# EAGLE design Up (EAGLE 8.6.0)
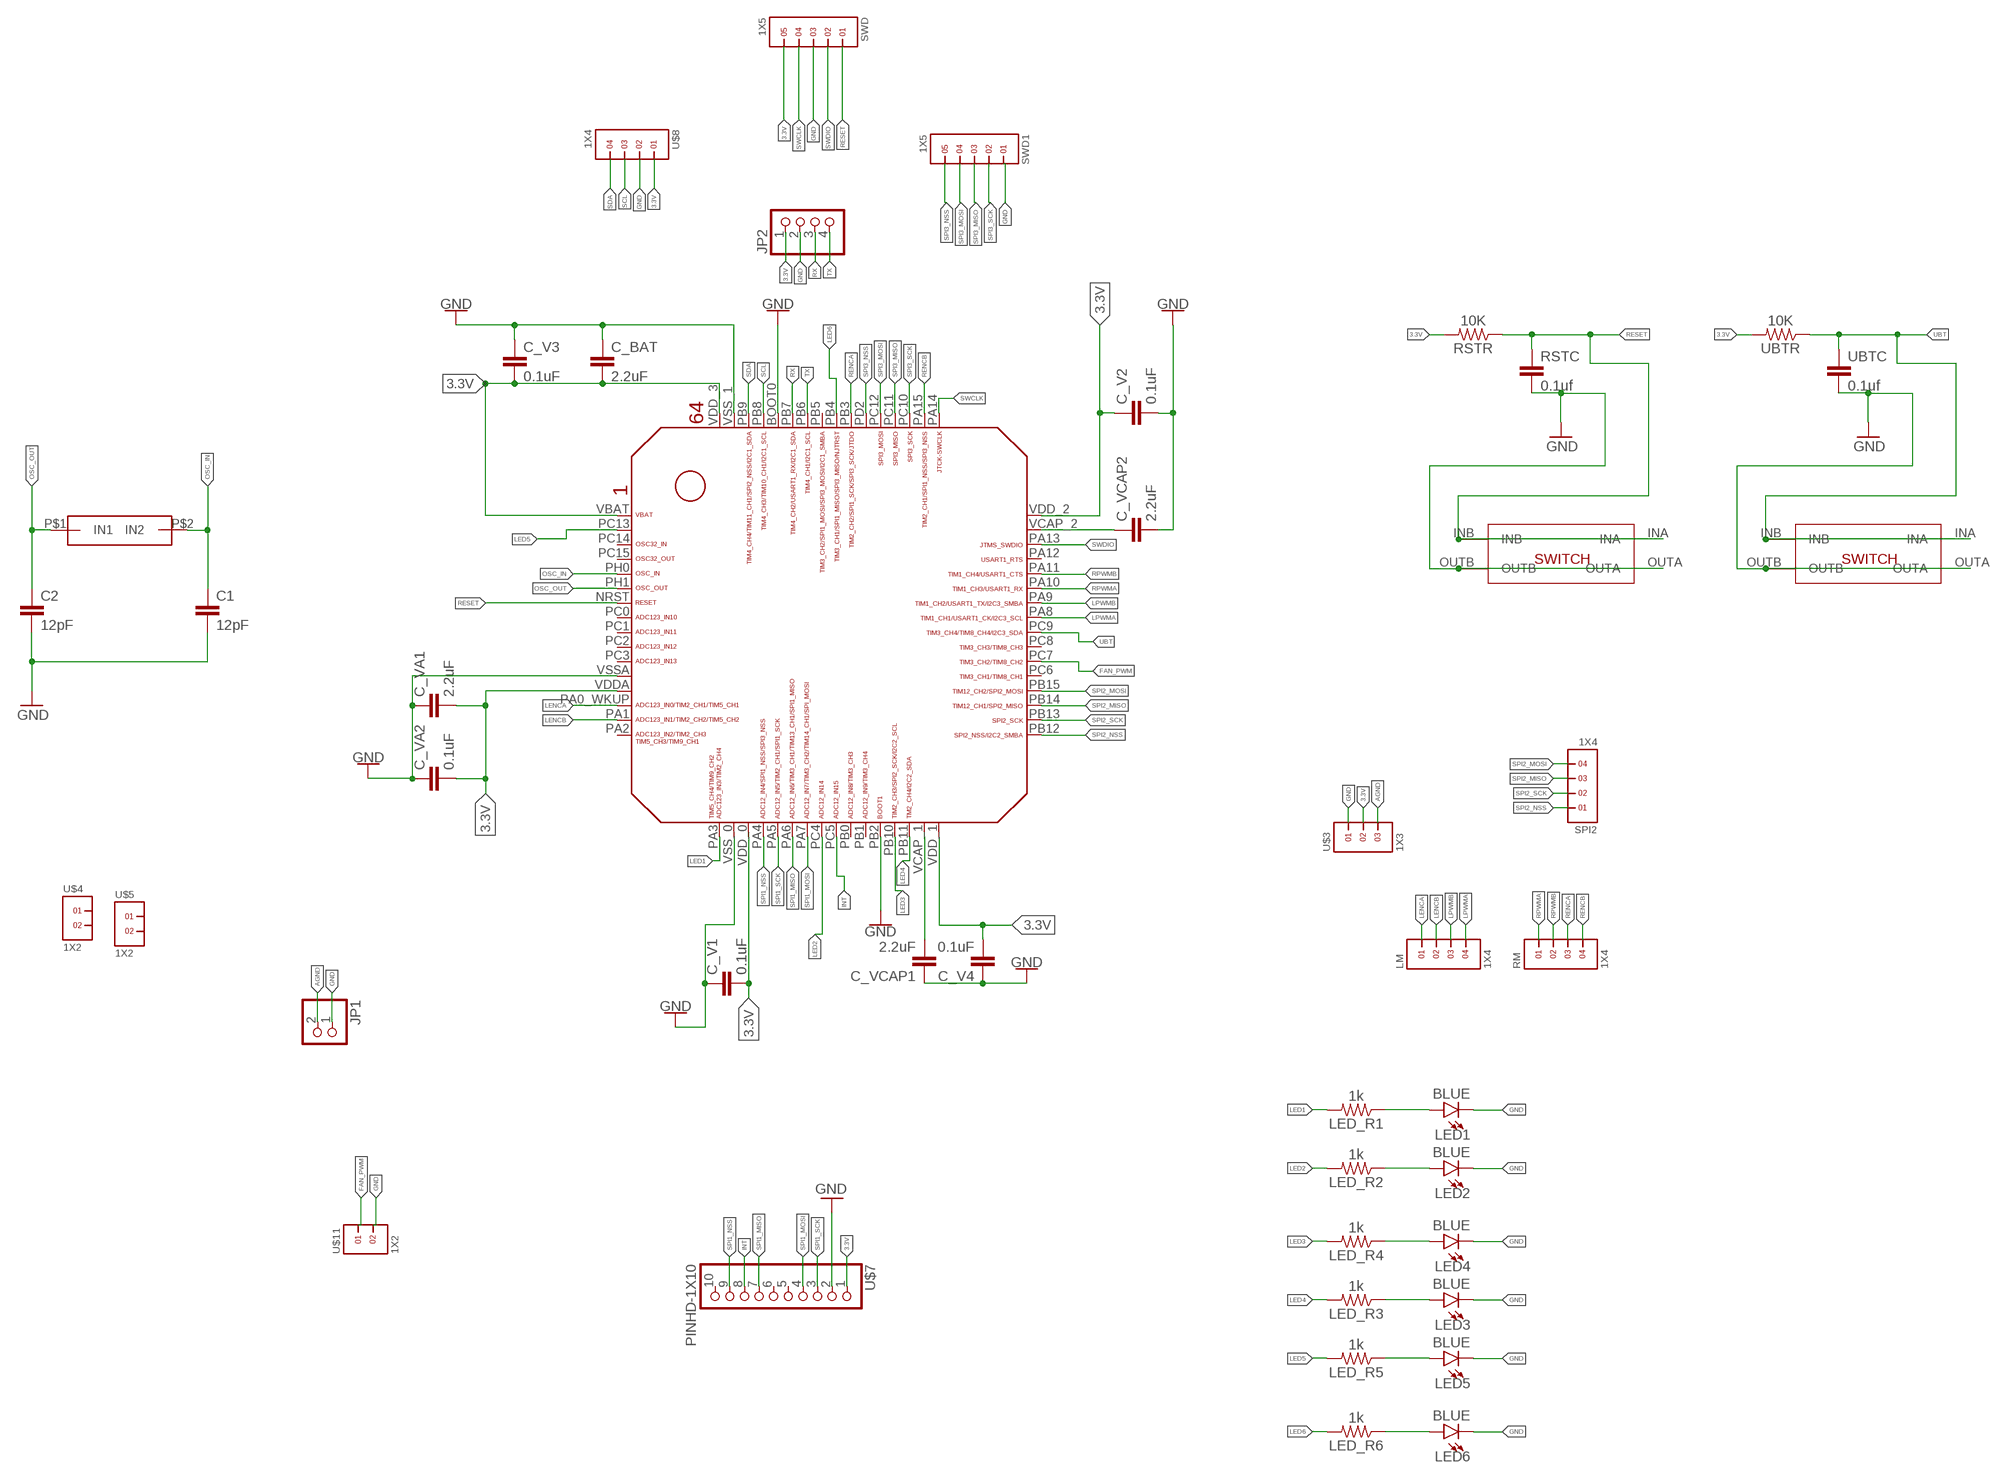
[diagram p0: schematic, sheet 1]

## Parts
C1  12pF  22PF-0603-50V-5%  [0603]
C2  12pF  22PF-0603-50V-5%  [0603]
C_BAT  2.2uF  22UF-0805-6.3V-20%  [0805]
C_V1  0.1uF  22UF-0805-6.3V-20%  [0805]
C_V2  0.1uF  22UF-0805-6.3V-20%  [0805]
C_V3  0.1uF  22UF-0805-6.3V-20%  [0805]
C_V4  0.1uF  22UF-0805-6.3V-20%  [0805]
C_VA1  2.2uF  22UF-0805-6.3V-20%  [0805]
C_VA2  0.1uF  22UF-0805-6.3V-20%  [0805]
C_VCAP1  2.2uF  22UF-0805-6.3V-20%  [0805]
C_VCAP2  2.2uF  22UF-0805-6.3V-20%  [0805]
CX5032GA  OSC  [OSC]
JP1  PINHD-1X2  [1X02]
JP2  PINHD-1X4  [1X04]
LED1  BLUE  LED-BLUE1206  [LED-1206]
LED2  BLUE  LED-BLUE1206  [LED-1206]
LED3  BLUE  LED-BLUE1206  [LED-1206]
LED4  BLUE  LED-BLUE1206  [LED-1206]
LED5  BLUE  LED-BLUE1206  [LED-1206]
LED6  BLUE  LED-BLUE1206  [LED-1206]
LED_R1  1k  0.75OHM-0805-1/4W-1%  [0805]
LED_R2  1k  0.75OHM-0805-1/4W-1%  [0805]
LED_R3  1k  0.75OHM-0805-1/4W-1%  [0805]
LED_R4  1k  0.75OHM-0805-1/4W-1%  [0805]
LED_R5  1k  0.75OHM-0805-1/4W-1%  [0805]
LED_R6  1k  0.75OHM-0805-1/4W-1%  [0805]
LM  1X4  [1X4]
RM  1X4  [1X4]
RSTC  0.1uf  22UF-0805-6.3V-20%  [0805]
RSTR  10K  0.75OHM-0805-1/4W-1%  [0805]
SPI2  1X4  [1X4]
SWD  1X5  [1X5]
SWD1  1X5  [1X5]
U$1  STM32F405/415_LQFP64  [STM32F405/415_LQFP64]
U$3  1X3  [1X3]
U$4  1X2  [1X2]
U$5  1X2  [1X2]
U$7  PINHD-1X10  [1X10-BIG]
U$8  1X4  [1X4]
U$9  4X4X1.5_SMD_SWITCH  [4X4X1.5_SMD_SWITCH]
U$10  4X4X1.5_SMD_SWITCH  [4X4X1.5_SMD_SWITCH]
U$11  1X2  [1X2]
UBTC  0.1uf  22UF-0805-6.3V-20%  [0805]
UBTR  10K  0.75OHM-0805-1/4W-1%  [0805]

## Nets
3.3V: C_BAT.2 C_V1.2 C_V2.1 C_V3.2 C_V4.2 C_VA1.2 C_VA2.2 JP2.1 RSTR.2 SWD.5 U$1.VBAT U$1.VDD_0 U$1.VDD_1 U$1.VDD_2 U$1.VDD_3 U$1.VDDA U$3.2 U$7.1 U$8.1 UBTR.2
AGND: JP1.2 U$3.3
FAN_PWM: U$1.PC7 U$11.1
GND: C1.2 C2.2 C_BAT.1 C_V1.1 C_V2.2 C_V3.1 C_V4.1 C_VA1.1 C_VA2.1 C_VCAP1.1 C_VCAP2.2 JP1.1 JP2.2 LED1.C LED2.C LED3.C LED4.C LED5.C LED6.C RSTC.2 SWD1.1 SWD.3 U$1.BOOT0 U$1.PB2 U$1.VSS_0 U$1.VSS_1 U$1.VSSA U$3.1 U$7.2 U$8.2 U$9.OUTA U$9.OUTB U$10.OUTA U$10.OUTB U$11.2 UBTC.2
INT: U$1.PC5 U$7.8
LED1: LED_R1.2 U$1.PA3
LED2: LED_R2.2 U$1.PC4
LED3: LED_R4.2 U$1.PB10
LED4: LED_R3.2 U$1.PB11
LED5: LED_R5.2 U$1.PC13
LED6: LED_R6.2 U$1.PB4
LENCA: LM.1 U$1.PA0_WKUP(PA0_AKUP)
LENCB: LM.2 U$1.PA1
LPWMA: LM.4 U$1.PA8
LPWMB: LM.3 U$1.PA9
N$1: LED3.A LED_R3.1
N$2: LED4.A LED_R4.1
N$3: LED5.A LED_R5.1
N$4: LED6.A LED_R6.1
N$5: LED2.A LED_R2.1
N$8: LED1.A LED_R1.1
OSC_IN: C1.1 CX5032GA.P$2(IN2) U$1.PH0
OSC_OUT: C2.1 CX5032GA.P$1(IN1) U$1.PH1
RENCA: RM.3 U$1.PB3
RENCB: RM.4 U$1.PA15
RESET: RSTC.1 RSTR.1 SWD.1 U$1.NRST U$9.INA U$9.INB
RPWMA: RM.1 U$1.PA10
RPWMB: RM.2 U$1.PA11
RX: JP2.3 U$1.PB7
SCL: U$1.PB8 U$8.3
SDA: U$1.PB9 U$8.4
SPI1_MISO: U$1.PA6 U$7.7
SPI1_MOSI: U$1.PA7 U$7.4
SPI1_NSS: U$1.PA4 U$7.9
SPI1_SCK: U$1.PA5 U$7.3
SPI2_MISO: SPI2.3 U$1.PB14
SPI2_MOSI: SPI2.4 U$1.PB15
SPI2_NSS: SPI2.1 U$1.PB12
SPI2_SCK: SPI2.2 U$1.PB13
SPI3_MISO: SWD1.3 U$1.PC11
SPI3_MOSI: SWD1.4 U$1.PC12
SPI3_NSS: SWD1.5 U$1.PD2
SPI3_SCK: SWD1.2 U$1.PC10
SWCLK: SWD.4 U$1.PA14
SWDIO: SWD.2 U$1.PA13
TX: JP2.4 U$1.PB6
UBT: U$1.PC9 U$10.INA U$10.INB UBTC.1 UBTR.1
VCAP_1: C_VCAP1.2 U$1.VCAP_1
VCAP_2: C_VCAP2.1 U$1.VCAP_2
Unconnected: U$1.PA2 U$1.PA12 U$1.PB0 U$1.PB1 U$1.PB5 U$1.PC0 U$1.PC1 U$1.PC2 U$1.PC3 U$1.PC6 U$1.PC8 U$1.PC14 U$1.PC15 U$4.1 U$4.2 U$5.1 U$5.2 U$7.5 U$7.6 U$7.10

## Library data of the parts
C1 C2 = SparkFun-Capacitors:22PF: 22pF ceramic capacitors; PROD_ID: CAP-07876; VALUE: 22pF
C_BAT C_V1-C_V4 C_VA1 C_VA2 C_VCAP1 C_VCAP2 RSTC UBTC = SparkFun-Capacitors:22UF: 22µF ceramic capacitors; PROD_ID: CAP-08402; VALUE: 22uF
CX5032GA = Cristal Oscillator:OSC
JP1 = pinhead:PINHD-1X2: PIN HEADER
JP2 = pinhead:PINHD-1X4: PIN HEADER
LED1-LED6 = SparkFun-LED:LED-BLUE: Blue SMD LED; PROD_ID: DIO-09911
LED_R1-LED_R6 RSTR UBTR = SparkFun-Resistors:0.75OHM: 0.75Ω resistor; PROD_ID: RES-08474; VALUE: 0.75
LM RM SPI2 U$8 = headers(2mm):1X4
SWD SWD1 = headers(2mm):1X5
U$1 = STM32F405RG:STM32F405/415_LQFP64
U$3 = headers(2mm):1X3
U$4 U$5 U$11 = headers(2mm):1X2
U$7 = adafruit:PINHD-1X10: Pin header 1x10 0.1" spacing With round pins
U$9 U$10 = 4X4X1.5_SMD_SWITCH:4X4X1.5_SMD_SWITCH

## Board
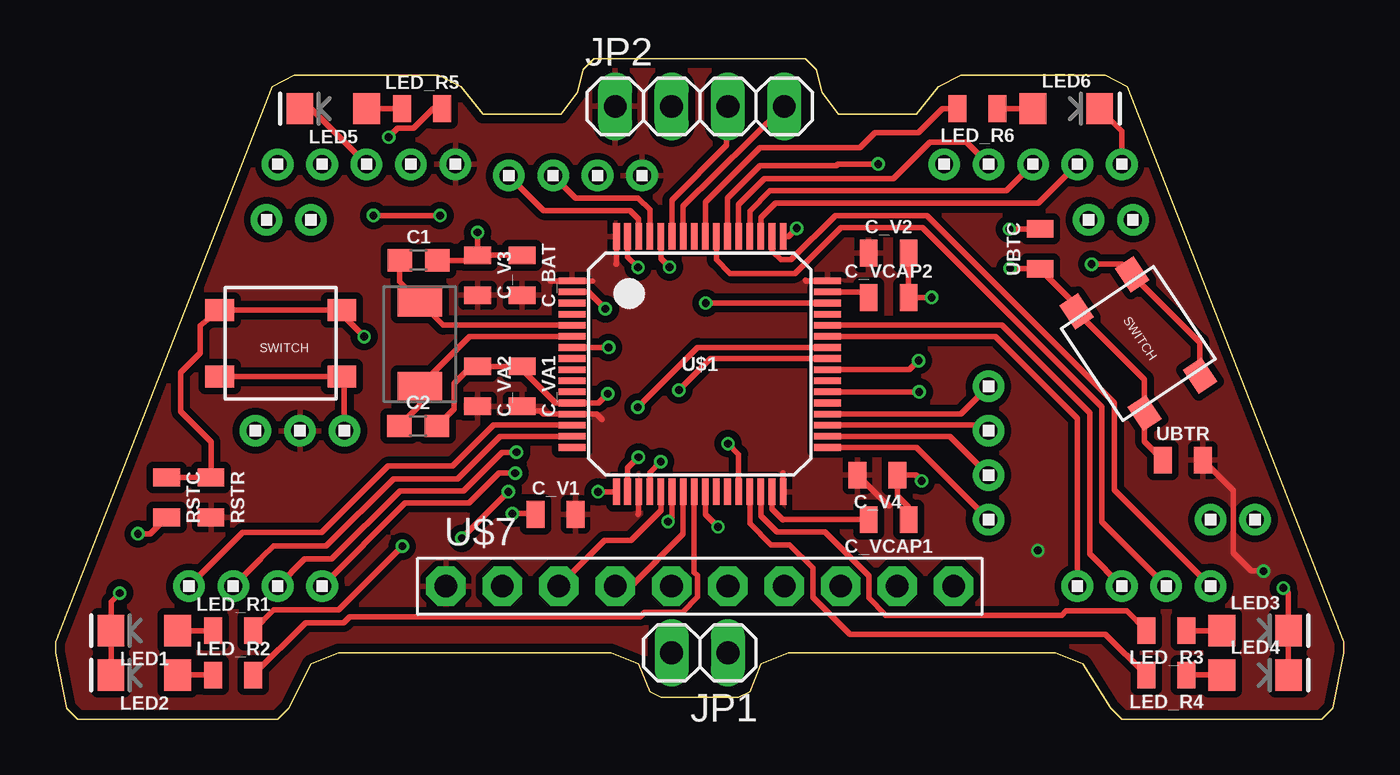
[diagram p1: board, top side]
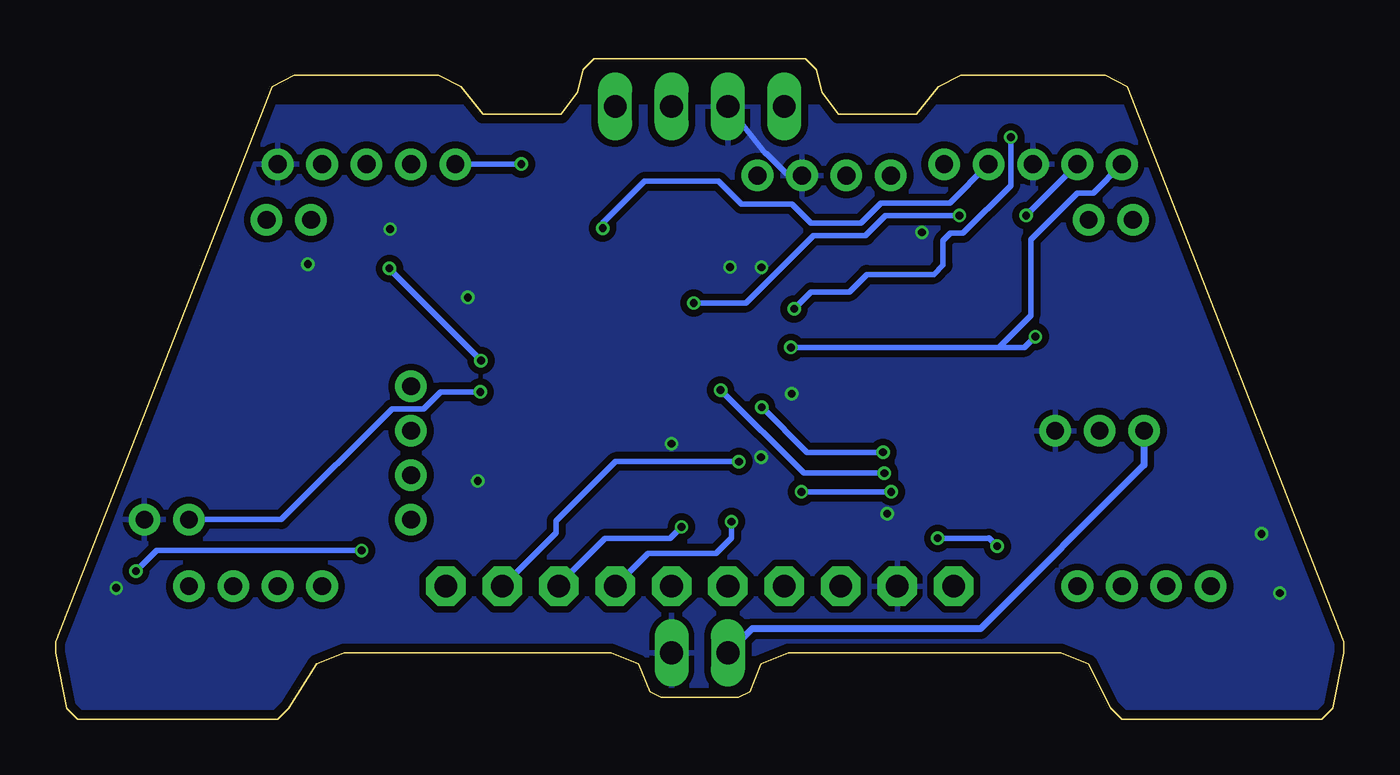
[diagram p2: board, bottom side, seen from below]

Size 58 x 29.75 mm. Coordinates in mm from the lower left corner, seen from the top.
Outline: 47.25,29 40.75,29 39.75,28.5 38.75,27.25 35.25,27.25 34.5,28.25 34.25,29.25 33.75,29.75 24.25,29.75 23.75,29.25 23.5,28.25 22.75,27.25 19.25,27.25 18.25,28.5 17.25,29 10.75,29 9.75,28.5 0,3.5 0,3 0.5,0.5 1,0 10,0 10.5,0.5 11.5,2.5 12.75,3 25,3 26.25,2.5 26.75,1.25 27.25,1 30.75,1 31.25,1.25 31.75,2.5 33,3 45,3 46.25,2.5 47.5,0.5 48,0 57,0 57.5,0.5 58,3 58,3.5 48.25,28.5 47.25,29
Copper layers (1*16): Top 0.035559375mm / dielectric 1.6mm / Bottom 0.035559375mm
Design rules "oshpark-2layer *": minimum track width 6mil, minimum drill 10mil, track to track 6mil, track to pad 6mil, pad to pad 6mil, via to via 6mil, smd to smd 6mil, copper to edge 15mil, drill to drill 6mil, minimum pad ring 5mil, minimum via ring 5mil, stop-mask expansion 2.5mil, vias tented up to drill 12mil, thermal gap 10mil

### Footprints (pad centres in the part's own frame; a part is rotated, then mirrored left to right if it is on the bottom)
0603 = smd 1.1 x 1: 1 -0.85,0; 2 0.85,0
0805 = smd 0.8 x 1.2: 1 -0.9,0; 2 0.9,0
OSC = smd 1.3 x 2: P$1 0,0.1; P$2 3.8,0.1
1X02 = drill 1.016 long: 1 -1.27,0; 2 1.27,0
1X04 = drill 1.016 long: 1 -3.81,0; 2 -1.27,0; 3 1.27,0; 4 3.81,0
LED-1206 = smd 1.2 x 1.4: A -1.5,0; C 1.5,0
1X4 = drill 0.8 pad 1.422: 1 -3,0; 2 -1,0; 3 1,0; 4 3,0
1X5 = drill 0.8 pad 1.422: 1 -4,0; 2 -2,0; 3 0,0; 4 2,0; 5 4,0
STM32F405/415_LQFP64 = smd 0.3 x 1.2: BOOT0 -1.75,5.75; PA3 -3.75,-5.75; PA4 -2.25,-5.75; PA5 -1.75,-5.75; PA6 -1.25,-5.75; PA7 -0.75,-5.75; PA14 3.75,5.75; PA15 3.25,5.75; PB0 0.75,-5.75; PB1 1.25,-5.75; PB2 1.75,-5.75; PB3 0.75,5.75; PB4 0.25,5.75; PB5 -0.25,5.75; PB6 -0.75,5.75; PB7 -1.25,5.75; PB8 -2.25,5.75; PB9 -2.75,5.75; PB10 2.25,-5.75; PB11 2.75,-5.75; PC4 -0.25,-5.75; PC5 0.25,-5.75; PC10 2.75,5.75; PC11 2.25,5.75; PC12 1.75,5.75; PD2 1.25,5.75; VCAP_1 3.25,-5.75; VDD_0 -2.75,-5.75; VDD_1 3.75,-5.75; VDD_3 -3.75,5.75; VSS_0 -3.25,-5.75; VSS_1 -3.25,5.75 | smd 1.2 x 0.3: NRST -5.75,0.75; PA0_WKUP -5.75,-2.75; PA1 -5.75,-3.25; PA2 -5.75,-3.75; PA8 5.75,0.25; PA9 5.75,0.75; PA10 5.75,1.25; PA11 5.75,1.75; PA12 5.75,2.25; PA13 5.75,2.75; PB12 5.75,-3.75; PB13 5.75,-3.25; PB14 5.75,-2.75; PB15 5.75,-2.25; PC0 -5.75,0.25; PC1 -5.75,-0.25; PC2 -5.75,-0.75; PC3 -5.75,-1.25; PC6 5.75,-1.75; PC7 5.75,-1.25; PC8 5.75,-0.75; PC9 5.75,-0.25; PC13 -5.75,3.25; PC14 -5.75,2.75; PC15 -5.75,2.25; PH0 -5.75,1.75; PH1 -5.75,1.25; VBAT -5.75,3.75; VCAP_2 5.75,3.25; VDD_2 5.75,3.75; VDDA -5.75,-2.25; VSSA -5.75,-1.75
1X3 = drill 0.8 pad 1.422: 1 -2,0; 2 0,0; 3 2,0
1X2 = drill 0.8 pad 1.422: 1 -1,0; 2 1,0
1X10-BIG = drill 1.016 pad 1.778 octagon: 1 -11.43,0; 2 -8.89,0; 3 -6.35,0; 4 -3.81,0; 5 -1.27,0; 6 1.27,0; 7 3.81,0; 8 6.35,0; 9 8.89,0; 10 11.43,0
4X4X1.5_SMD_SWITCH = smd 1.3 x 1: INA -2.75,-1.5; INB 2.75,-1.5; OUTA -2.75,1.5; OUTB 2.75,1.5

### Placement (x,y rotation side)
C1  16.34,20.67 0 top
C2  16.32,13.21 0 top
C_BAT  21,20 270 top
C_V1  22.51,9.23 0 top
C_V2  37.5,21 0 top
C_V3  19,20 270 top
C_V4  37,11 180 top
C_VA1  21,15 270 top
C_VA2  19,15 270 top
C_VCAP1  37.5,9 180 top
C_VCAP2  37.5,19 0 top
CX5032GA  16.5,15 90 top
JP1  29,3 180 top
JP2  29,27.61 0 top
LED1  4,4 180 top
LED2  4,2 180 top
LED3  54,4 0 top
LED4  54,2 0 top
LED5  12.5,27.5 180 top
LED6  45.5,27.5 0 top
LED_R1  8,4 0 top
LED_R2  8,2 0 top
LED_R3  50,4 180 top
LED_R4  50,2 180 top
LED_R5  16.5,27.5 0 top
LED_R6  41.5,27.5 180 top
LM  9,6 0 top
RM  49,6 0 top
RSTC  5,10 270 top
RSTR  7,10 270 top
SPI2  42,12 90 top
SWD  14,25 0 top
SWD1  44,25 180 top
U$1  29,16 0 top
U$3  11,13 180 top
U$4  10.5,22.5 0 top
U$5  47.5,22.5 0 top
U$7  29,6 0 top
U$8  23.4,24.49 180 top
U$9  10.14,16.94 180 top
U$10  48.74,16.92 303.8 top
U$11  53,9 0 top
UBTC  44.32,21.19 90 top
UBTR  50.75,11.68 0 top

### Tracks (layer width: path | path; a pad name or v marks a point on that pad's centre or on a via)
3.3V  (via drill 0.35)
  Top 0.254: C_VA1.2 21.21,13.89 21.84,13.89 21.98,13.75 U$1.VDDA 24.36,13.75 24.6,13.51 | 26.22,9.24 26.25,9.27 U$1.VDD_0 | U$1.VDD_1 32.75,11.09 32.74,11.1 | U$1.VDD_2 33.79,19.75 33.76,19.78 | 24.17,19.74 24.16,19.75 U$1.VBAT 22.28,19.75 22.27,19.76 | U$1.VDD_3 25.25,20.51 25.24,20.5 | C_V4.2 37.4,9.7 37.42,9.7 37.51,9.61 37.54,9.61 | UBTR.2 53.01,10.32 53.01,8.59 53.01,7.5 53.83,6.68 v54.38,6.68
  Bottom 0.254: v54.38,6.68 53.45,7.61 v44.22,7.61
  pour Top (isolate 0.305): -4.12,-4.71 62.31,-4.71 62.31,31.86 -4.13,31.86
AGND
  Bottom 0.305: U$3.3 9,11.45 16.36,4.09 26.64,4.09 JP1.2
FAN_PWM  (via drill 0.35)
  Top 0.254: U$1.PC7 v38.88,14.75
  Bottom 0.254: v38.88,14.75 40.66,14.75 41.42,13.99 41.59,13.99 42.85,13.99 47.84,9 U$11.1
GND  (via drill 0.35)
  Top 0.254: C_V2.2 C_VCAP2.2 v39.44,19 | C_VCAP1.1 38.4,9.57 37.9,10.07 C_V4.1 38.73,11 v38.99,10.74 | C2.2 17.93,13.97 17.93,15.13 18.7,15.9 C_VA2.1 C_VA1.1 21,15.75 22.5,14.25 U$1.VSSA 24.44,14.25 v24.86,14.67 | C1.2 18.77,20.67 C_V3.1 | C_V3.1 C_BAT.1 | U$1.VSS_1 25.75,20.83 v26.22,20.36 | U$1.BOOT0 27.25,20.76 v27.64,20.37 | U$1.VSS_0 25.75,11.32 v26.24,11.81 | C_V1.1 21.57,9.27 v20.56,9.27 | U$1.PB2 30.75,11.94 v30.27,12.42 | C_V3.1 v19,21.93 | UBTC.2 v42.95,22.09 v42.94,22.08 | v46.64,20.5 48,20.5 U$10.OUTA 51.52,16.98 U$10.OUTB | U$9.OUTB U$9.OUTA 13,15.16 U$3.1 | RSTC.2 4.26,8.36 v3.71,8.36 | LED2.C LED1.C 2.5,5.3 v2.89,5.69 | LED4.C LED3.C 55.5,5.69 v55.27,5.92 | SWD.3 11.5,27.5 LED5.C | SWD1.1 48,26.5 LED6.C
  Bottom 0.254: JP2.2 26.04,25.48 25.99,25.48 25,24.49 U$8.2
  pour Bottom (isolate 0.305): -0.43,2.98 -0.43,27.57 57.55,27.57 58.44,27.57 58.44,2.81 58.44,-0.99 -0.21,-0.99 -0.44,-0.99 -0.44,2.99
INT  (via drill 0.35)
  Top 0.254: U$1.PC5 29.25,9.24 v29.82,8.67
  Bottom 0.254: v29.82,8.67 30.33,8.16 33.26,8.16 35.35,6.07 U$7.8
LED1  (via drill 0.35)
  Top 0.254: v15.61,7.8 12.74,4.93 9.83,4.93 LED_R1.2 | v20.38,10.25 v18.29,8.16 | U$1.PA3 v24.42,10.25
  Bottom 0.254: v15.61,7.8 15.98,8.17 15.99,8.16 v18.29,8.16 | v24.42,10.25 v20.38,10.25
LED2
  Top 0.254: U$1.PC4 28.75,6.63 28.9,6.48 28.9,5.52 28.21,4.83 26.52,4.83 26.32,4.63 13.24,4.63 12.96,4.35 11.25,4.35 LED_R2.2
LED3
  Top 0.254: U$1.PB10 31.25,8.82 32.2,7.87 33.05,7.87 34.09,6.83 34.09,5.5 35.75,3.84 47.26,3.84 LED_R4.2
LED4
  Top 0.254: U$1.PB11 31.75,9.17 32.48,8.44 34.63,8.44 36.61,6.46 36.61,5.47 37.37,4.71 37.37,4.69 45.29,4.69 45.48,4.88 48.22,4.88 LED_R3.2
LED5  (via drill 0.35)
  Top 0.254: v15,26.22 15.4,26.62 16.12,26.62 16.99,27.5 LED_R5.2 | U$1.PC13 23.99,19.25 v24.75,18.49
  Bottom 0.254: v15,26.22 15,24.04 17.15,21.89 17.72,21.89 18.05,21.56 18.05,20.45 18.46,20.04 21.48,20.04 22.27,19.25 23.99,19.25 v24.75,18.49
LED6
  Top 0.254: U$1.PB4 29.25,23.29 31.71,25.75 36.22,25.75 36.89,26.42 38.83,26.42 39.92,27.5 LED_R6.2 40.41,27.5
LENCA
  Top 0.254: U$1.PA0_WKUP 19.72,13.25 17.88,11.41 14.97,11.41 11.99,8.43 8.43,8.43 LM.1
LENCB
  Top 0.254: U$1.PA1 20.01,12.75 18.09,10.83 15.21,10.83 12.19,7.81 9.81,7.81 9.31,7.31 9.24,7.24 LM.2
LPWMA  (via drill 0.35)
  Top 0.254: U$1.PA8 29.48,16.25 v28.06,14.83 | LM.4 15.74,9.74 18.62,9.74 19.97,11.09 v20.69,11.09
  Bottom 0.254: v20.69,11.09 24.32,11.09 v28.06,14.83
LPWMB  (via drill 0.35)
  Top 0.254: LM.3 11.22,7.22 12.43,7.22 15.51,10.3 18.37,10.3 20.1,12.03 v20.75,12.03 | v26.21,14.06 28.9,16.75 U$1.PA9
  Bottom 0.254: v26.21,14.06 24.18,12.03 v20.75,12.03
N$1
  Top 0.254: LED_R3.1 LED3.A
N$2
  Top 0.254: LED_R4.1 LED4.A
N$3
  Top 0.254: LED5.A LED_R5.1
N$4
  Top 0.254: LED_R6.1 LED6.A
N$5
  Top 0.254: LED_R2.1 LED2.A
N$8
  Top 0.254: LED_R1.1 LED1.A
OSC_IN
  Top 0.254: C1.1 15.49,19.71 CX5032GA.P$2 17.45,17.75 U$1.PH0
OSC_OUT
  Top 0.254: C2.1 16.4,14.14 CX5032GA.P$1 18.65,17.25 U$1.PH1
RENCA
  Top 0.254: RM.3 47.1,8.9 47.1,14.06 39.02,22.15 35.34,22.15 33.28,20.08 30.37,20.08 29.75,20.7 U$1.PB3
RENCB
  Top 0.254: U$1.PA15 32.25,21.1 32.65,20.7 33.11,20.7 35.1,22.69 39.23,22.69 47.66,14.26 47.66,10.34 RM.4
RESET  (via drill 0.35)
  Top 0.254: U$1.NRST v24.9,16.75 | v13.89,17.24 12.72,18.41 U$9.INA U$9.INB 6.51,17.73 6.51,16.49 5.64,15.62 5.64,13.86 7,12.5 RSTR.1 RSTC.1
  Bottom 0.254: v24.9,16.75 15.54,16.75 | 15.54,16.75 14.1,18.19 14.1,21.61 12,23.71 11.29,23.71 SWD.1 | 15.54,16.75 14.38,16.75 v13.89,17.24
RPWMA
  Top 0.254: U$1.PA10 42.31,17.25 46,13.56 RM.1
RPWMB
  Top 0.254: U$1.PA11 42.6,17.75 46.55,13.8 46.55,7.45 RM.2
RX
  Top 0.254: U$1.PB7 27.75,23.39 30.21,25.85 JP2.3
SCL
  Top 0.254: U$8.3 23.41,23.48 26.23,23.48 26.75,22.96 U$1.PB8
SDA
  Top 0.254: U$8.4 21.97,22.92 25.85,22.92 26.25,22.52 U$1.PB9
SPI1_MISO  (via drill 0.35)
  Top 0.254: U$1.PA6 27.75,9.09 v27.57,8.91
  Bottom 0.254: v27.57,8.91 27.57,8.18 28.27,7.48 31.33,7.48 U$7.7
SPI1_MOSI
  Top 0.254: U$1.PA7 28.25,8.35 25.9,6 U$7.4
SPI1_NSS  (via drill 0.35)
  Top 0.254: U$1.PA4 26.75,11.12 v27.24,11.61
  Bottom 0.254: U$7.9 37.87,6 35.46,8.41 35.46,8.94 32.79,11.61 v27.24,11.61
SPI1_SCK
  Top 0.254: U$7.3 24.71,8.06 25.9,8.06 27.25,9.41 U$1.PA5
SPI2_MISO
  Top 0.254: SPI2.3 41.75,13.25 U$1.PB14
SPI2_MOSI
  Top 0.254: U$1.PB15 40.75,13.75 SPI2.4
SPI2_NSS
  Top 0.254: U$1.PB12 38.75,12.25 SPI2.1
SPI2_SCK
  Top 0.254: U$1.PB13 40.25,12.75 SPI2.2
SPI3_MISO
  Top 0.254: U$1.PC11 31.25,22.89 32.17,23.81 42.81,23.81 SWD1.3
SPI3_MOSI
  Top 0.254: U$1.PC12 30.75,23.19 31.92,24.36 37.73,24.36 39.36,25.99 40.41,25.99 40.41,25.98 41.02,25.98 SWD1.4
SPI3_NSS  (via drill 0.35)
  Top 0.254: U$1.PD2 30.25,23.48 31.71,24.94 35.15,24.94 35.22,25.01 v37.03,25.01
  Bottom 0.254: v37.03,25.01 SWD1.5
SPI3_SCK
  Top 0.254: U$1.PC10 31.75,22.6 32.4,23.25 44.25,23.25 SWD1.2
SWCLK  (via drill 0.35)
  Top 0.254: U$1.PA14 33,21.75 v33.37,22.12
  Bottom 0.254: v33.37,22.12 33.37,22.34 31.48,24.23 28.15,24.23 27.12,23.2 24.85,23.2 24,22.35 21.74,22.35 20.84,23.25 17.75,23.25 SWD.4
SWDIO  (via drill 0.35)
  Top 0.254: U$1.PA13 v29.27,18.75 | v17.31,22.69 v14.31,22.69
  Bottom 0.254: v14.31,22.69 SWD.2 | v29.27,18.75 26.92,18.75 23.89,21.78 21.54,21.78 20.63,22.69 v17.31,22.69
TX
  Top 0.254: U$1.PB6 28.25,23.11 JP2.4
UBT  (via drill 0.35)
  Top 0.254: U$1.PC9 38.44,15.75 v38.85,16.16 | v42.97,20.31 44.3,20.31 UBTC.1 45.96,18.65 U$10.INA 49.02,15.31 U$10.INB 49.02,12.51 UBTR.1
  Bottom 0.254: v38.85,16.16 42.97,20.28 v42.97,20.31
VCAP_1
  Top 0.254: U$1.VCAP_1 32.25,9.49 32.75,8.99 32.76,9 C_VCAP1.2
VCAP_2
  Top 0.254: U$1.VCAP_2 36.35,19.25 C_VCAP2.1

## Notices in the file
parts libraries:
SparkFun-PowerSymbols: Licensing: Creative Commons ShareAlike 4.0 International - https://creativecommons.org/licenses/by-sa/4.0
